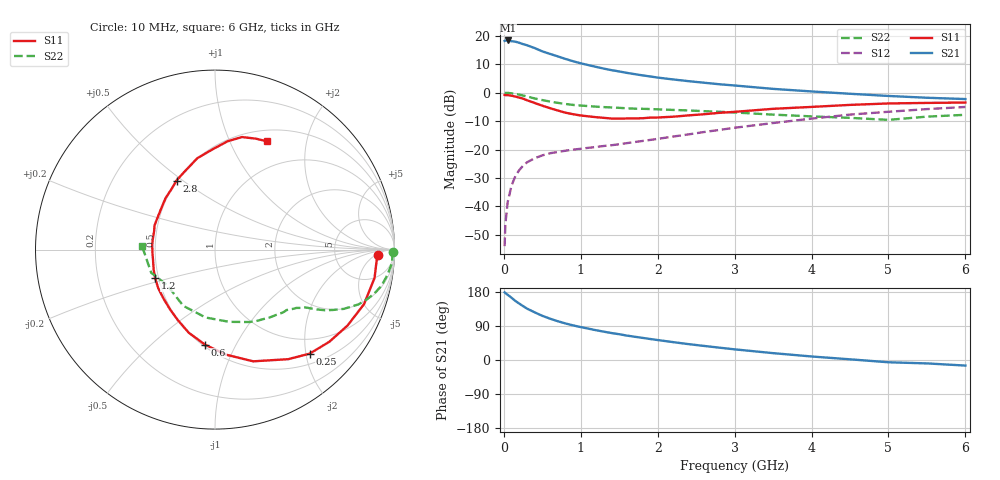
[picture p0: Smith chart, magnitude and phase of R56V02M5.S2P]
! SIEMENS Small Signal Semiconductors
! BFR183
! Si NPN RF Bipolar Junction Transistor in SOT23
! VCE = 6 V  IC = 2.5 mA
! Common Emitter S-Parameters:  May  1996
# GHz  S  MA  R  50
!  f  S11  S21  S12  S22
! GHz  MAG  ANG  MAG  ANG  MAG  ANG  MAG  ANG
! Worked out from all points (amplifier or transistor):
!   36 points, 10 MHz to 6 GHz, reference 50 ohm
!   highest |S21| = 18.3 dB at 50 MHz (marker M1)
!   |S21| within 3 dB of that: start of sweep to 428.3 MHz
!   unconditionally stable (mu >= 1): 1.336 GHz to 2.797 GHz
!   at 250 MHz: K = 0.26, MSG = 21.4 dB, |S12| = -25.7 dB
!   at 1.4 GHz: K = 1.03, MAG = 12.2 dB, |S12| = -18.5 dB
!   at 6 GHz: K = 0.88, MSG = 1.4 dB, |S12| = -5.0 dB
!   S11 on the Smith chart (normalised r, x): 10 MHz: 18, -7; 250 MHz: 0.69, -2.07; 600 MHz: 0.51, -0.76; 1.2 GHz: 0.48, -0.18; 2.8 GHz: 0.50, +0.47; 6 GHz: 0.64, +1.39
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0.01  0.9083 -2.0  8.096 178.6  0.002 88.6  0.9942 -0.8
0.02  0.9026 -4.0  8.185 176.6  0.0049 83.0  0.9888 -1.6
0.05  0.9029 -10.1  8.251 172.0  0.0119 84.0  0.9893 -4.2
0.15  0.8511 -29.8  7.856 155.8  0.034 72.9  0.9498 -12.2
0.2  0.8182 -38.9  7.508 148.9  0.0434 68.9  0.9201 -15.5
0.25  0.7836 -47.7  7.116 142.2  0.052 64.8  0.8887 -18.3
0.3  0.7346 -56.2  6.806 135.8  0.0594 61.4  0.8558 -20.9
0.4  0.658 -71.1  6.067 125.8  0.0702 55.9  0.7901 -24.7
0.5  0.5886 -84.0  5.306 116.6  0.0788 51.9  0.7383 -27.1
0.6  0.5325 -96.0  4.784 109.1  0.0859 49.1  0.6964 -29.0
0.7  0.4854 -107.6  4.339 102.4  0.0904 47.6  0.6612 -30.3
0.8  0.444 -117.8  3.911 96.5  0.0952 46.4  0.6312 -31.4
0.9  0.4172 -126.8  3.558 91.4  0.0995 46.6  0.6075 -32.2
1.1  0.3826 -145.6  3.041 82.7  0.1071 46.9  0.579 -34.1
1.2  0.3697 -154.6  2.831 78.5  0.1108 47.4  0.5664 -35.0
1.6  0.351 175.7  2.22 64.4  0.1294 50.7  0.5301 -39.1
2.2  0.377 142.8  1.703 47.2  0.1688 54.5  0.4962 -47.6
2.8  0.4405 119.1  1.403 32.6  0.2206 54.2  0.4609 -59.5
3.5  0.5189 100.9  1.163 18.1  0.2919 49.4  0.4102 -78.9
4.5  0.608 83.3  0.954 1.8  0.4106 38.4  0.3598 -119.5
5.5  0.6586 69.8  0.812 -9.0  0.5131 24.5  0.3782 -160.0
6  0.6691 64.4  0.77 -14.7  0.5592 15.7  0.4073 177.1
